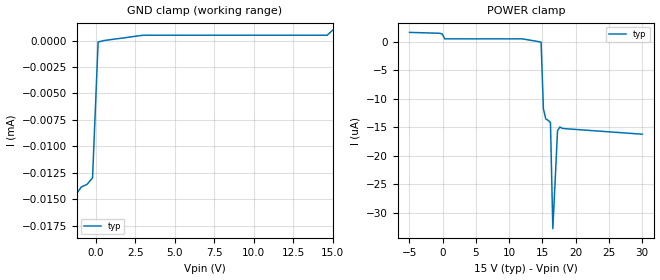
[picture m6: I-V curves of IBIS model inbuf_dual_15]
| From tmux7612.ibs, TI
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| inbuf_dual_15
[Model]   inbuf_dual_15
Model_type   Input
Vinl = 0.8
Vinh = 1.3
|   typ   min   max
C_comp   2.533030e-12   NA   NA
[Voltage Range]   15   NA   NA
[Temperature Range]   27   NA   NA
[Power Clamp Reference]   15   NA   NA
[GND Clamp Reference]   0   NA   NA
[GND Clamp]
|   Voltage   I(typ)   I(min)   I(max)
-20V      -3.924A    NA         NA
-15.76V   -278.6uA   NA         NA
-15.4V    -16.28uA   NA         NA
-2.677V   -15.01uA   NA         NA
-2.323V   -15.24uA   NA         NA
-1.97V    -22.57uA   NA         NA
-1.616V   -39.83uA   NA         NA
-1.263V   -14.58uA   NA         NA
-202mV    -12.98uA   NA         NA
151.5mV   -138.9nA   NA         NA
14.65V    500.4nA    NA         NA
15V       976nA      NA         NA
[POWER Clamp]
|   Voltage   I(typ)   I(min)   I(max)
-5V       1.635uA    NA         NA
-404mV    1.479uA    NA         NA
303mV     500.4nA    NA         NA
11.97V    498.2nA    NA         NA
14.8V     -78.02nA   NA         NA
15.15V    -11.81uA   NA         NA
15.51V    -13.57uA   NA         NA
16.21V    -14.21uA   NA         NA
16.57V    -32.83uA   NA         NA
17.27V    -15.63uA   NA         NA
17.63V    -14.98uA   NA         NA
30V       -16.24uA   NA         NA
